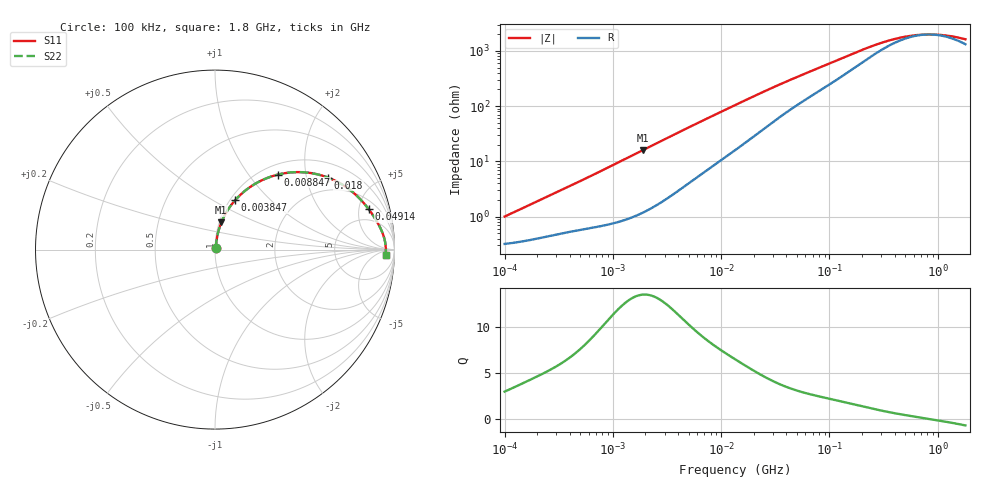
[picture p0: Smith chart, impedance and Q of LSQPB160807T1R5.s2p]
! LSQPB160807T1R5  S-PARAMETER MODEL  ( General Type )
! Model Generated by TAIYO YUDEN Corporation (http://www.ty-top.com)
! Version 1.0
! TAIYO YUDEN Control No. 110308NG25SB-FKC
! Copyright(c) 2011 TAIYO YUDEN CO.,LTD. All Rights Reserved.
! Product Description (link to TY-COMPAS)
! https://ds.yuden.co.jp/TYCOMPAS/or/detail?pn=LSQPB160807T1R5M&u=M
! Products Name : Inductors
! Characteristics :
!  Inductance : 1.5 uH , SRF(min) : 600 MHz , DC Resistance(max) : 0.364 Ohm
!  Rated Current : Saturation :440 mA , Temp Rise : 590 mA (40 degC)
!  Case Size : 1.6 x 0.8 / 0.063 x 0.031 [mm/inch] , Thickness : 0.7 / 0.028 [mm/inch]
!  (Conditions: Temperature = 25 degC , DC Bias Current/Voltage = 0A / 0V)
! External Node Assignments :
!  1  o---GGG---o  2
! GND o---------o GND
! Frequency Range : 0.1MHz  -  1800MHz  [ 402 STEP ]
# MHz S RI R 50
! Freq[MHz].  S11 Real  S11 Imag  S21 Real  S21 Imag  S12 Real  S12 Imag  S22 Real  S22 Imag
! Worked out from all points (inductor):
!   401 points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, 100 kHz to 1.8 GHz, reference 50 ohm
!   read as one part in series: L = 1.5 uH near 105 kHz
!   highest Q = 13.5 at 1.891 MHz (marker M1), where L = 1.34 uH
!   self-resonance near 820.2 MHz
!   S11 on the Smith chart (normalised r, x): 100 kHz: 1.01, +0.02; 3.847 MHz: 1.06, +0.64; 8.847 MHz: 1.18, +1.40; 18 MHz: 1.48, +2.69; 49.14 MHz: 3.03, +6.31; 1.8 GHz: 27, -19
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0.1  0.00327 0.00942  0.9967 -0.00942  0.9967 -0.00942  0.00327 0.00942
0.516129  0.00773 0.0443  0.9923 -0.0443  0.9923 -0.0443  0.00773 0.0443
1.050184  0.0153 0.0872  0.9847 -0.0872  0.9847 -0.0872  0.0153 0.0872
1.890522  0.0354 0.1516  0.9646 -0.1516  0.9646 -0.1516  0.0354 0.1516
2.66389  0.0617 0.2053  0.9383 -0.2053  0.9383 -0.2053  0.0617 0.2053
3.846706  0.1118 0.2748  0.8882 -0.2748  0.8882 -0.2748  0.1118 0.2748
5.833619  0.2081 0.357  0.7919 -0.357  0.7919 -0.357  0.2081 0.357
8.84682  0.3497 0.4178  0.6503 -0.4178  0.6503 -0.4178  0.3497 0.4178
11.02886  0.4376 0.431  0.5624 -0.431  0.5624 -0.431  0.4376 0.431
13.41641  0.5174 0.4286  0.4826 -0.4286  0.4826 -0.4286  0.5174 0.4286
18.00091  0.6298 0.4013  0.3702 -0.4013  0.3702 -0.4013  0.6298 0.4013
22.99727  0.7088 0.3625  0.2912 -0.3625  0.2912 -0.3625  0.7088 0.3625
28.66948  0.7656 0.3217  0.2344 -0.3217  0.2344 -0.3217  0.7656 0.3217
49.1428  0.8561 0.2253  0.1439 -0.2253  0.1439 -0.2253  0.8561 0.2253
69.24595  0.8905 0.1754  0.1095 -0.1754  0.1095 -0.1754  0.8905 0.1754
118.6955  0.9245 0.1134  0.0755 -0.1134  0.0755 -0.1134  0.9245 0.1134
218.9722  0.9432 0.0626  0.0568 -0.0626  0.0568 -0.0626  0.9432 0.0626
357.3983  0.9491 0.0343  0.0509 -0.0343  0.0509 -0.0343  0.9491 0.0343
542.0029  0.9512 0.0158  0.0488 -0.0158  0.0488 -0.0158  0.9512 0.0158
802.0705  0.952 0.000832  0.048 -0.000832  0.048 -0.000832  0.952 0.000832
1186.925  0.952 -0.0141  0.048 0.0141  0.048 0.0141  0.952 -0.0141
1800  0.9512 -0.0324  0.0488 0.0324  0.0488 0.0324  0.9512 -0.0324
